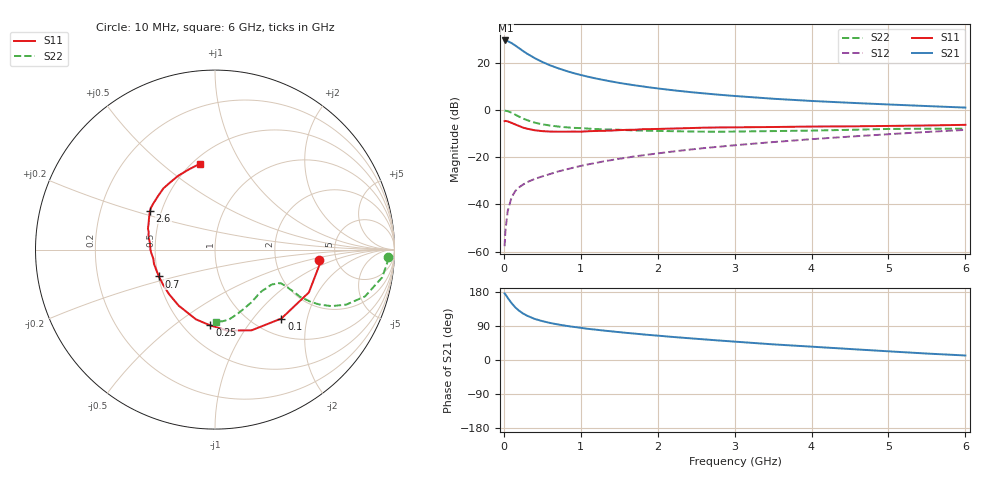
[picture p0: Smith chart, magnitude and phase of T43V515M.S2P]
! Infineon Technologies  Discrete & RF Semiconductors
! BFR182T
! Si NPN RF Bipolar Junction Transistor in SC75
! VCE = 3.5 V  IC = 15 mA
! Common Emitter S-Parameters:  October  1999
# GHz  S  MA  R  50
!  f  S11  S21  S12  S22
! GHz  MAG  ANG  MAG  ANG  MAG  ANG  MAG  ANG
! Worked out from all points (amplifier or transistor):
!   36 points, 10 MHz to 6 GHz, reference 50 ohm
!   highest |S21| = 29.5 dB at 20 MHz (marker M1)
!   |S21| within 3 dB of that: start of sweep to 186.1 MHz
!   unconditionally stable (mu >= 1): 782.7 MHz to 3.684 GHz
!   at 250 MHz: K = 0.56, MSG = 28.3 dB, |S12| = -31.6 dB
!   at 1.4 GHz: K = 1.09, MAG = 14.8 dB, |S12| = -21.2 dB
!   at 6 GHz: K = 0.84, MSG = 4.7 dB, |S12| = -8.4 dB
!   S11 on the Smith chart (normalised r, x): 10 MHz: 3.64, -0.65; 100 MHz: 1.31, -1.41; 250 MHz: 0.67, -0.68; 700 MHz: 0.50, -0.17; 2.6 GHz: 0.43, +0.23; 6 GHz: 0.54, +0.68
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0.01  0.5803 -5.9  29.74 175.7  0.0013 72.3  0.9637 -2.6
0.02  0.5878 -8.5  29.79 173.5  0.0027 95.0  0.9649 -3.8
0.05  0.575 -24.5  28.86 164.0  0.0072 83.1  0.9444 -9.4
0.1  0.5331 -46.1  26.21 150.2  0.014 73.8  0.8759 -17.3
0.15  0.4937 -65.6  23.19 138.6  0.0193 67.8  0.7935 -22.7
0.2  0.4569 -81.2  20.33 129.7  0.0231 64.5  0.7211 -25.9
0.25  0.4227 -93.8  17.8 122.7  0.0263 62.6  0.6583 -27.7
0.3  0.4028 -105.3  15.72 117.1  0.0294 61.8  0.6113 -28.6
0.4  0.372 -123.0  12.61 108.5  0.0346 61.5  0.54 -29.0
0.5  0.3566 -135.9  10.44 102.6  0.0392 62.7  0.4986 -28.2
0.6  0.3493 -146.0  8.861 97.8  0.0439 64.1  0.4688 -27.8
0.7  0.3466 -154.4  7.713 93.9  0.0495 64.9  0.4474 -27.3
0.9  0.3491 -166.9  6.093 87.6  0.0597 67.1  0.419 -27.1
1.1  0.3552 -176.7  5.049 82.1  0.0707 68.3  0.4033 -27.7
1.3  0.3624 176.0  4.313 77.6  0.0817 68.9  0.3896 -28.8
1.6  0.3801 167.2  3.532 71.5  0.0977 69.4  0.3746 -31.1
2.2  0.4047 155.5  2.622 60.8  0.1319 69.0  0.3558 -37.9
2.6  0.4223 149.0  2.25 54.5  0.1558 68.0  0.3478 -43.0
3.5  0.436 136.4  1.733 41.3  0.209 64.7  0.3572 -55.9
4.5  0.4499 123.9  1.422 29.0  0.273 59.8  0.3802 -71.1
5.5  0.47 108.0  1.212 17.0  0.3429 53.9  0.4015 -84.1
6  0.4848 100.2  1.125 11.9  0.379 50.2  0.4012 -89.4
